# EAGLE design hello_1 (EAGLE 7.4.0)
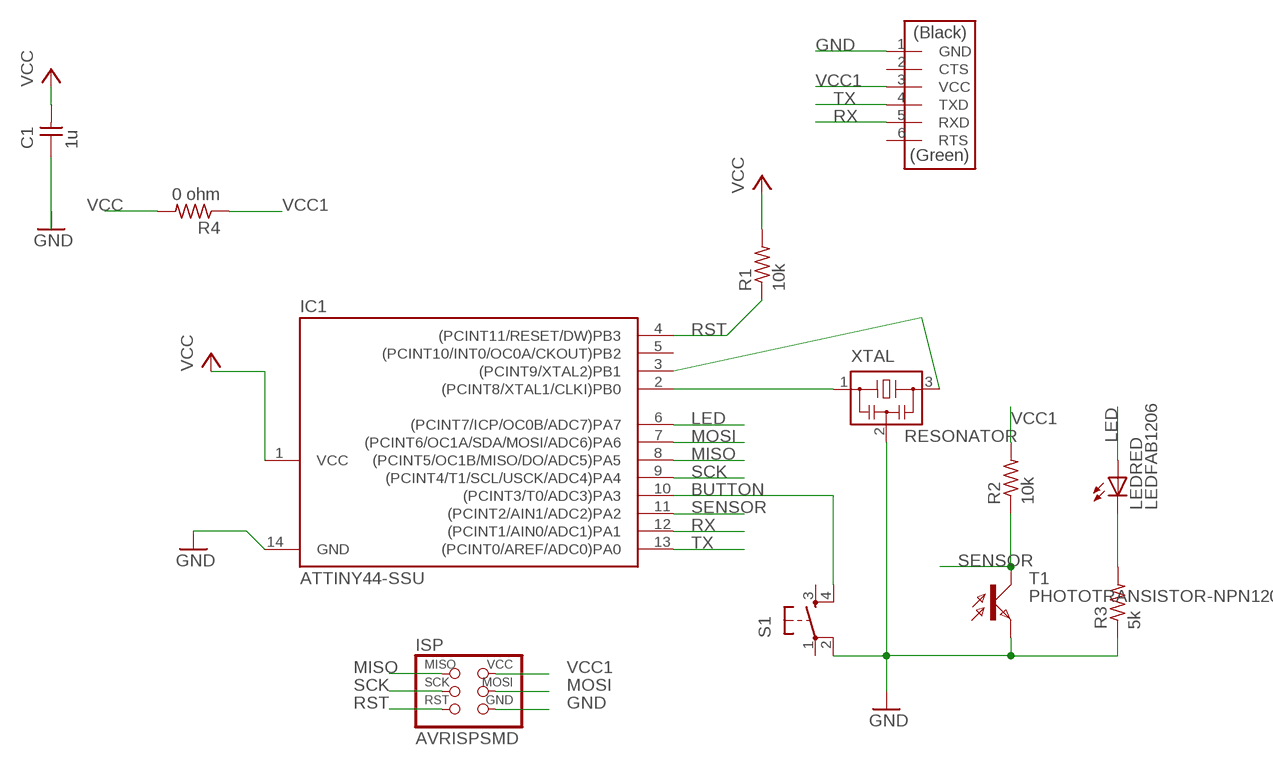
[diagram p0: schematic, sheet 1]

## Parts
C1  1u  CAP-UNPOLARIZEDFAB  [C1206FAB]
IC1  ATTINY44-SSU  [SOIC14]
ISP  AVRISPSMD  [2X03SMD]
LEDRED  LEDFAB1206  [LED1206FAB]
R1  10k  RES-US1206FAB  [R1206FAB]
R2  10k  RES-US1206FAB  [R1206FAB]
R3  5k  RES-US1206FAB  [R1206FAB]
R4  0 ohm  RES-US1206FAB  [R1206FAB]
S1  6MM_SWITCH6MM_SWITCH  [6MM_SWITCH]
T1  PHOTOTRANSISTOR-NPN1206  [OP1206]
U$1  FTDI-SMD-HEADER  [1X06SMD]
XTAL  RESONATOR  [EFOBM]

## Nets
BUTTON: IC1.10((PCINT3/T0/ADC3)PA3) S1.4(S1)
GND: IC1.14(GND) ISP.6(GND) R3.1 S1.2(P1) T1.EMITTER(E) U$1.1(GND) XTAL.2
LED: IC1.6((PCINT7/ICP/OC0B/ADC7)PA7) LEDRED.1(A)
MISO: IC1.8((PCINT5/OC1B/MISO/DO/ADC5)PA5) ISP.1(MISO)
MOSI: IC1.7((PCINT6/OC1A/SDA/MOSI/ADC6)PA6) ISP.4(MOSI)
N$1: IC1.2((PCINT8/XTAL1/CLKI)PB0) XTAL.1
N$2: IC1.3((PCINT9/XTAL2)PB1) XTAL.3
N$3: LEDRED.2(C) R3.2
N$4: C1.1
RST: IC1.4((PCINT11/RESET/DW)PB3) ISP.5(RST) R1.1
RX: IC1.12((PCINT1/AIN0/ADC1)PA1) U$1.5(RXD)
SCK: IC1.9((PCINT4/T1/SCL/USCK/ADC4)PA4) ISP.3(SCK)
SENSOR: IC1.11((PCINT2/AIN1/ADC2)PA2) R2.1 T1.COLLECTOR(C)
TX: IC1.13((PCINT0/AREF/ADC0)PA0) U$1.4(TXD)
VCC: C1.2 IC1.1(VCC) R1.2 R4.2
VCC1: ISP.2(VCC) R2.2 R4.1 U$1.3(VCC)
Unconnected: IC1.5((PCINT10/INT0/OC0A/CKOUT)PB2) S1.1(P) S1.3(S) U$1.2(CTS) U$1.6(RTS)

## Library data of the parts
C1 = fab:CAP-UNPOLARIZED
IC1 = fab:ATTINY44
ISP = fab:AVRISP
LEDRED = fab:LED: LED
R1-R4 = fab:RES-US: Resistor (US Symbol)
S1 = ng:6MM_SWITCH: OMRON SWITCH
T1 = fab:PHOTOTRANSISTOR-NPN
U$1 = fab:FTDI-SMD-HEADER
XTAL = fab:RESONATOR

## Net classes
0 default: width 0.4 mm, clearance 0.4 mm

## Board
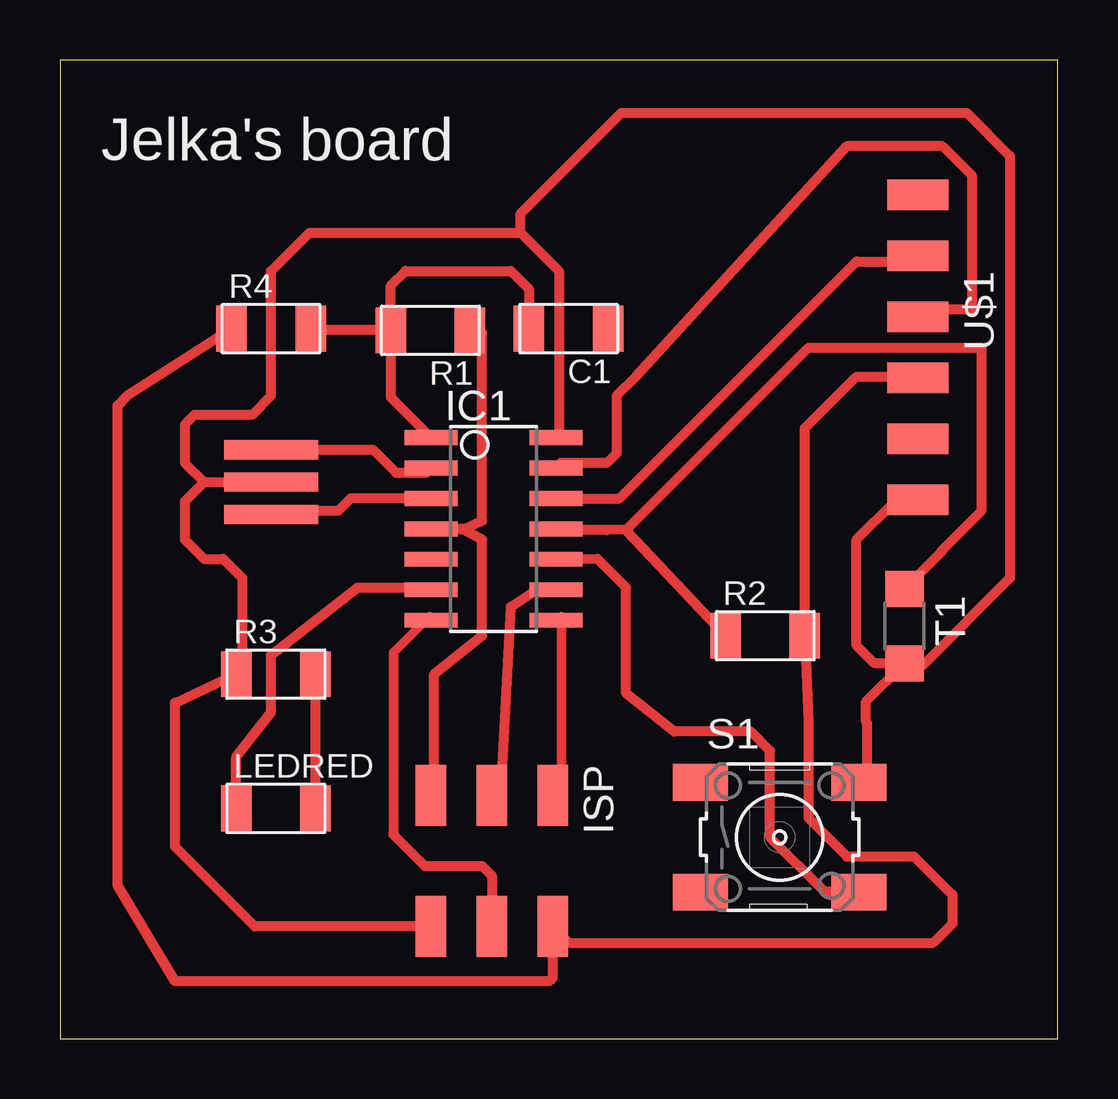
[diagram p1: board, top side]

Size 41.6 x 40.8 mm. Coordinates in mm from the lower left corner, seen from the top.
Outline: 0,0 41.6,0 41.6,40.8 0,40.8 0,0
Copper layers (1*16): Top 0.035mm / dielectric 1.5mm / Bottom 0.035mm
Design rules "default *": minimum track width 0.3mm, minimum drill 0.8mm, track to track 0.4mm, track to pad 0.4mm, pad to pad 0.4mm, via to via 8mil, smd to smd 8mil, copper to edge 40mil, drill to drill 8mil, minimum pad ring 10mil, minimum via ring 8mil, stop-mask expansion 4mil, vias tented up to drill 0mil, thermal gap 10mil

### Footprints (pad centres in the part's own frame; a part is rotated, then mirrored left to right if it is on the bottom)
C1206FAB = smd 1.27 x 1.905: 1 -1.651,0; 2 1.651,0
SOIC14 = smd 0.61 x 2.21: 1 -3.81,-2.603; 2 -2.54,-2.603; 3 -1.27,-2.603; 4 0,-2.603; 5 1.27,-2.603; 6 2.54,-2.603; 7 3.81,-2.603; 8 3.81,2.603; 9 2.54,2.603; 10 1.27,2.603; 11 0,2.603; 12 -1.27,2.603; 13 -2.54,2.603; 14 -3.81,2.603
2X03SMD = smd 2.54 x 1.27: 1 -2.54,2.54; 2 2.92,2.54; 3 -2.54,0; 4 2.92,0; 5 -2.54,-2.54; 6 2.92,-2.54
LED1206FAB = smd 1.27 x 1.905: 1 -1.651,0; 2 1.651,0
R1206FAB = smd 1.27 x 1.905: 1 -1.651,0; 2 1.651,0
6MM_SWITCH = smd 2.286 x 1.524: 1 -3.302,2.286; 2 3.302,2.286; 3 -3.302,-2.286; 4 3.302,-2.286
OP1206 = smd 1.5 x 1.6: COLLECTOR -1.55,0; EMITTER 1.55,0
1X06SMD = smd 2.54 x 1.27: 1 0,6.35; 2 0,3.81; 3 0,1.27; 4 0,-1.27; 5 0,-3.81; 6 0,-6.35
EFOBM = smd 0.8 x 3.9: 1 -1.35,0; 2 0,0; 3 1.35,0

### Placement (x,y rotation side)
C1  21.2,29.6 180 top
IC1  18.07,21.25 270 top
ISP  18,7.6 270 top
LEDRED  9,9.6 0 top
R1  15.44,29.53 180 top
R2  29.4,16.8 0 top
R3  9,15.2 0 top
R4  8.8,29.6 0 top
S1  30,8.4 0 top
T1  35.2,17.2 270 top
U$1  35.76,28.82 180 top
XTAL  8.8,23.2 270 top

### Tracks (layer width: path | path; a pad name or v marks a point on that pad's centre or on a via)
BUTTON
  Top 0.4: 20.9,20.1 IC1.10
  Top 0.406: S1.4 31.89,6.11 29.6,8.4 29.6,12 28.8,12.8 25.6,12.8 23.6,14.4 23.6,18.8 22.4,20 IC1.10
GND
  Top 0.4: 20.9,25.1 IC1.14
  Top 0.406: ISP.6 8.12,4.68 4.8,8 4.8,14 R3.1 7.6,15.45 7.6,19.2 6.8,20 6,20 5.2,20.8 5.2,22.4 6,23.2 | 19.2,33.6 20.8,32 20.8,25.19 IC1.14 20.81,25.2 | 19.2,33.6 10.4,33.6 8.8,32 8.8,26.8 8,26 5.6,26 5.2,25.6 5.2,24 6,23.2 | S1.2 33.65,11.03 33.65,13.15 33.6,13.2 33.6,14.05 T1.EMITTER | 19.2,33.6 19.2,34.4 23.4,38.6 37.8,38.6 39.6,36.8 39.6,19.2 36,15.6 35.25,15.6 T1.EMITTER | T1.EMITTER 33.95,15.65 33.2,16.4 33.2,20.8 34.8,22.4 35.69,22.4 U$1.1 | 6,23.2 XTAL.2
LED
  Top 0.4: 15.4,18.6 IC1.6
  Top 0.406: 7.2,9.75 arc90 LEDRED.1 7.35,11.75 8.8,13.6 8.8,16 12.4,18.8 15.38,18.8 IC1.6
MISO
  Top 0.4: IC1.8 20.9,17.6 20.9,10.6 ISP.1
MOSI
  Top 0.4: 13.9,8.6 13.9,16.1 15.4,17.6 IC1.7 | 17.9,5.1 ISP.4
  Top 0.406: 13.9,8.6 13.9,8.5 15.2,7.2 17.6,7.2 18,6.8 ISP.4
N$1
  Top 0.406: XTAL.1 13.05,24.55 14,23.6 15.28,23.6 IC1.2
N$2
  Top 0.406: IC1.3 12.12,22.52 11.6,22 8.95,22 XTAL.3
N$3
  Top 0.406: LEDRED.2 R3.2
RST
  Top 0.406: ISP.5 15.6,10.28 15.6,15.2 17.6,16.8 17.6,20.8 16.75,21.25 IC1.4 16.85,21.25 17.6,21.6 17.6,29.42 R1.1
RX
  Top 0.406: IC1.12 23.32,22.52 33.2,32.4 35.53,32.4 U$1.5
SCK
  Top 0.4: 20.4,18.6 IC1.9 | 18.4,10.6 ISP.3
  Top 0.406: 18.4,10.6 18.8,18 20,18.8 IC1.9
SENSOR
  Top 0.406: IC1.11 21.6,21.23 | 21.6,21.23 22.8,21.2 | 23.6,21.2 21.6,21.23 | 23.6,21.2 R2.1 | T1.COLLECTOR 36.75,20.3 36.75,20.35 38.4,22 38.4,28.8 31.2,28.8 23.6,21.2
TX
  Top 0.406: 35.11,30.09 35.2,30 35.29,30.09 U$1.4 36.07,30.4 38,30.4 38,36 36.8,37.2 32.8,37.2 24,27.6 23.2,26.8 23.2,24.4 22.8,24 20.88,24 IC1.13
VCC
  Top 0.4: 15.4,25.1 IC1.1
  Top 0.406: R1.2 10.52,29.53 R4.2 | R1.2 13.79,26.74 IC1.1 | R1.2 13.79,31.39 14.4,32 18.8,32 19.55,31.25 C1.2
VCC1
  Top 0.406: R4.1 2.8,26.8 2.4,26.4 2.4,6.4 4.8,2.4 20.4,2.4 20.54,2.54 ISP.2 21.22,4 36.4,4 37.2,4.8 37.2,6 35.6,7.6 32.8,7.6 31.2,9.2 31.2,13.2 R2.2 31.05,25.45 33.2,27.6 35.71,27.6 U$1.3

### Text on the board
tPlace: Jelka's board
